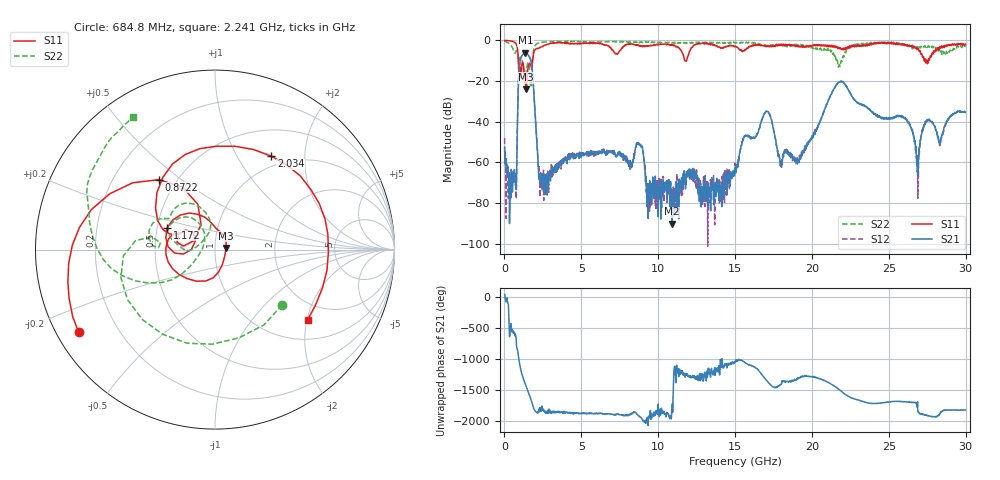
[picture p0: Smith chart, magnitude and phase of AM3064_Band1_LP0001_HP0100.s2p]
# Hz S DB R 50.0
!freq dBS11 angS11 dBS21 angS21 dBS12 angS12 dBS22 angS22
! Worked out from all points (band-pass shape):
!   1600 points, 10 MHz to 29.98 GHz, reference 50 ohm
!   highest |S21| = -6.09 dB at 1.36 GHz (marker M1); lowest = -90.2 dB at 10.88 GHz (marker M2)
!   |S21| within 3 dB of the highest: 1.048 GHz to 1.684 GHz (636.3 MHz wide, 46.6 % of centre)
!   lowest |S11| = -24.1 dB at 1.416 GHz (marker M3), VSWR 1.13, Z = 56.6 + j1.05 ohm
!   |S11| at or under -10 dB: 901.9 MHz to 1.83 GHz (928.6 MHz wide, 68 % of centre); 11.75 GHz to 11.84 GHz (93.58 MHz wide, 0.793 % of centre); 27.48994 GHz to 27.56343 GHz (73.49 MHz wide, 0.267 % of centre)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
!   |S22| runs from -23.2 to -0.2 dB; largest |S21 - S12| = 0.0065
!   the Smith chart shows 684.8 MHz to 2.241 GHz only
!   S11 on the Smith chart (normalised r, x): 684.8 MHz: 0.06, -0.28; 872.2 MHz: 0.40, +0.42; 1.172 GHz: 0.57, +0.15; 2.034 GHz: 0.85, +1.41; 2.241 GHz: 1.50, -2.02
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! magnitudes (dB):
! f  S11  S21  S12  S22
! 10 MHz  -0.1  -53.0  -48.1  -0.2
! 684.8 MHz  -1.0  -65.7  -67.3  -6.3
! 872.2 MHz  -6.0  -31.3  -31.2  -7.0
! 1.172 GHz  -10.7  -7.2  -7.1  -10.3
! 1.36 GHz  -20.1  -6.1  -6.1  -18.2
! 1.416 GHz  -24.1  -6.2  -6.2  -14.9
! 2.034 GHz  -4.3  -41.1  -40.9  -2.1
! 2.241 GHz  -3.8  -65.9  -61.3  -1.2
! 5.015 GHz  -1.4  -55.2  -56.7  -0.7
! 8.745 GHz  -2.6  -51.2  -51.3  -1.1
! 9.344 GHz  -2.9  -87.6  -72.5  -0.9
! 10 GHz  -2.0  -86.8  -72.7  -0.9
! 10.88 GHz  -2.3  -90.2  -78.5  -1.2
! 15 GHz  -3.0  -64.5  -60.5  -1.3
! 17.03 GHz  -3.1  -34.8  -34.9  -2.6
! 17.95 GHz  -2.3  -61.8  -59.3  -2.1
! 19.99 GHz  -3.0  -47.5  -47.6  -3.4
! 21.83 GHz  -3.9  -20.3  -20.3  -13.0
! 25 GHz  -1.1  -38.3  -38.0  -1.1
! 26.87 GHz  -4.4  -63.3  -64.2  -3.3
! 27.47 GHz  -9.7  -39.0  -39.5  -2.7
! 29.98 GHz  -1.8  -35.4  -35.2  -3.1
